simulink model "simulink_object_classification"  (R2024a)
settings: Solver=FixedStepAuto  StartTime=0.0  StopTime=inf  RelTol=1e-3  EnableMultiTasking=on
undefined symbols (not defined in the file): uint
libraries: visionsources x2, visionsinks x2, deeplib x1, visiontextngfix x1

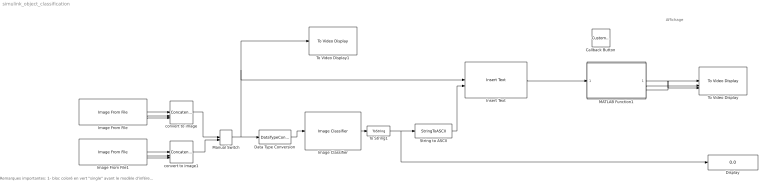
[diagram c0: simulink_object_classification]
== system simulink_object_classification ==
  note: Remarques importantes: 1- bloc coloré en vert "single" avant le modèle d'inférence (toujours le cas pour du DL) 2- bloc coloré en bleu clair: utiliser votre modèle sauvegardé en .mat et attention aux nomx des classes que vous devez avoir déclaré dans le workspace de MATLAB
  note: Affichage
  Callback Button : CustomCallbackButton  Configuration="{\"components\":[{\"name\":\"BackgroundImageComponent\",\"settings\":{\"image\":{\"size\":[0,0],\"src\":\"default\",\"srcOrientation\":\"Right\"},\"position\":[0,0,1,1]}},{\"name\":\"ButtonStateComponent\",\"settings\":{\"buttonType\":\"momentary\",\"clickFcn\":\"showExample('raspberrypi\\/ClassifyObjectsDeepLearningRaspberryPiHardwareExample')\",\"onValue\":1,\"position\":[0,0,1,1],\"pressDelay\":\"500\",\"pressFcn\":\"\",\"repeatInterval\":\"0\",\"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"  CustomBackgroundColor="{\"color\":[0.9568627451,0.9568627451,0.9568627451],\"show\":true}"
  Data Type Conversion : DataTypeConversion  OutDataTypeStr=single
  Display : Display
  Image Classifier : deeplib/Image Classifier  Network=Network from MAT-file  NetworkFunction=resnet50  NetworkFilePath=C:\work\PASS\Tonnerre\SI-IA-VigneNette-main\SI-IA-VigneNette-main\2-TransferLearning\monSqueeze.mat  NetworkClassesVariable=classNames  MiniBatchSize=128  ResizeInput=on  Classification=on  Predictions=off  ForceInterpretedSim=off  PredictMode=All probabilities and labels  K=5
  Image From File : visionsources/Image From File  Tag=vipblks_nd  FileName=C:\work\PASS\Tonnerre\SI-IA-VigneNette-main\SI-IA-VigneNette-main\2-TransferLearning\grape2classes\Grape___Esca\0ad02171-f9d0-4d0f-bdbd-36ac7674fafc___FAM_B.Msls 4356.JPG  Ts=1/30  imagePorts=Separate color signals  OutPortLabels=R|G|B  ImageDataType=Inherit from input image  sdImageDataType=uint(8)  Signed=on  WordLength=16  FractionLengthMode=User-defined  FractionLength=15
  Image From File1 : visionsources/Image From File  Tag=vipblks_nd  FileName=C:\work\PASS\Tonnerre\SI-IA-VigneNette-main\SI-IA-VigneNette-main\2-TransferLearning\grape2classes\Grape___healthy\0ca59865-f0d2-4863-b4d1-a6690de53a5a___Mt.N.V_HL 6025_90deg.JPG  Ts=1/30  imagePorts=Separate color signals  OutPortLabels=R|G|B  ImageDataType=Inherit from input image  sdImageDataType=uint(8)  Signed=on  WordLength=16  FractionLengthMode=User-defined  FractionLength=15
  Insert Text : visiontextngfix/Insert Text  inputType=Obsolete  theText='%s'  getTextLocFrom=Specify via dialog  textLoc=[1 1]  getTextColorFrom=Specify via dialog  textColor=[255,255,0]  getTextIntensityFrom=Specify via dialog  textIntensity=0  getTextOpacityFrom=Specify via dialog  textOpacity=1.0  dummyVar2=0  dummyVar3=0  dummyVar4=0  imagePorts=One multidimensional signal  isInputTransposed=on  fontFace=LucidaSansRegular  dummyVar1=0  blockFontSize=18  antiAliased=off
  MATLAB Function1 : MATLAB Function  TreatAsAtomicUnit=on
  Manual Switch : ManualSwitch  CurrentSetting=0
  String to ASCII : StringToASCII
  To String1 : ToString
  To Video Display : visionsinks/To Video Display  windowSizeMode=Normal  openAtMdlStart=on  fullScreen=off  videoWindowX=1467  videoWindowY=321  saveWindowSize=off  videoWindowWidth=256  videoWindowHeight=308  inputColorFormat=RGB  inputType=Obsolete  imagePorts=Separate color signals  OutputDevice=On-screen video monitor  dataOrg=Column-major  isWindowOpen=off
  To Video Display1 : visionsinks/To Video Display  windowSizeMode=Normal  openAtMdlStart=on  fullScreen=off  videoWindowX=536805376  videoWindowY=536805376  saveWindowSize=off  videoWindowWidth=256  videoWindowHeight=256  inputColorFormat=RGB  inputType=Obsolete  imagePorts=One multidimensional signal  OutputDevice=On-screen video monitor  dataOrg=Column-major  isWindowOpen=off
  convert to image : Concatenate  NumInputs=3  Mode=Multidimensional array  ConcatenateDimension=3
  convert to image1 : Concatenate  NumInputs=3  Mode=Multidimensional array  ConcatenateDimension=3
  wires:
  MATLAB Function1/2(g) -> To Video Display/2
  MATLAB Function1/3(b) -> To Video Display/3
  convert to image/1 -> Manual Switch/1
  To String1/1 -> Display/1, String to ASCII/1
  MATLAB Function1/1(r) -> To Video Display/1
  Image From File/3 -> convert to image/3
  Image From File/2 -> convert to image/2
  Image From File/1 -> convert to image/1
  Insert Text/1 -> MATLAB Function1/1(i)
  String to ASCII/1 -> Insert Text/2
  Image Classifier/1 -> To String1/1
  Image From File1/2 -> convert to image1/2
  Image From File1/3 -> convert to image1/3
  Image From File1/1 -> convert to image1/1
  Manual Switch/1 -> To Video Display1/1, Insert Text/1, Data Type Conversion/1
  convert to image1/1 -> Manual Switch/2
  Data Type Conversion/1 -> Image Classifier/1

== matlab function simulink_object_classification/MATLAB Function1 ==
function [r,g,b] = ImageToRGB(i)
%#codegen
r =i(:,:,1);
g =i(:,:,2);
b =i(:,:,3);
end
